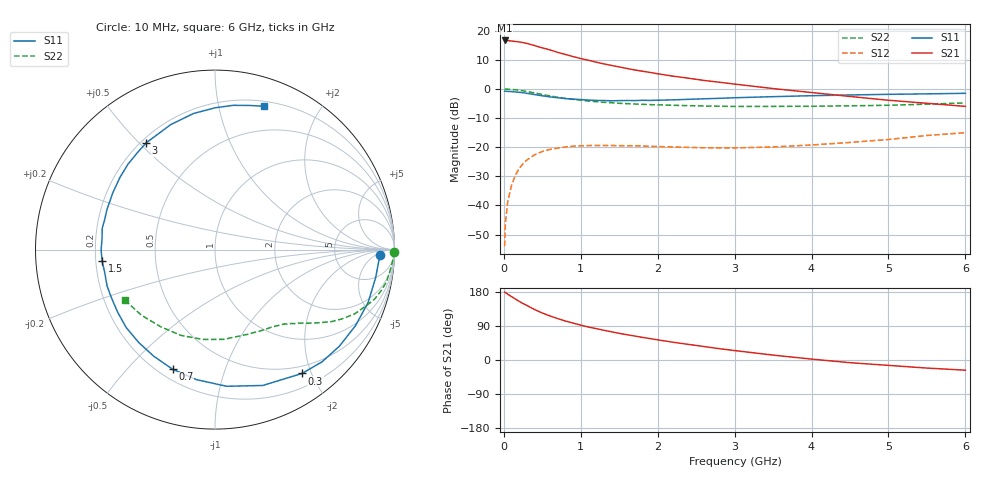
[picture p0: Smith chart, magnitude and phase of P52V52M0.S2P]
! SIEMENS Small Signal Semiconductors
! BFP183
! Si NPN RF Bipolar Junction Transistor in SOT143
! VCE = 2.5 V  IC = 2 mA
! Common Emitter S-Parameters:  March  1996
# GHz  S  MA  R  50
!  f  S11  S21  S12  S22
! GHz  MAG  ANG  MAG  ANG  MAG  ANG  MAG  ANG
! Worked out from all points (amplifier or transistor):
!   36 points, 10 MHz to 6 GHz, reference 50 ohm
!   highest |S21| = 16.7 dB at 10 MHz (marker M1)
!   |S21| within 3 dB of that: start of sweep to 565.9 MHz
!   unconditionally stable (mu >= 1): 2.092 GHz to 5.891 GHz
!   at 250 MHz: K = 0.12, MSG = 20.8 dB, |S12| = -25.7 dB
!   at 1.4 GHz: K = 0.68, MSG = 13.7 dB, |S12| = -19.4 dB
!   at 6 GHz: K = 0.98, MSG = 4.5 dB, |S12| = -15.0 dB
!   S11 on the Smith chart (normalised r, x): 10 MHz: 21, -8; 300 MHz: 0.39, -1.86; 700 MHz: 0.25, -0.68; 1.5 GHz: 0.23, -0.05; 3 GHz: 0.22, +0.52; 6 GHz: 0.25, +1.37
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0.01  0.9206 -1.8  6.819 179.0  0.002 88.4  0.999 -0.7
0.02  0.915 -3.9  6.79 178.0  0.0049 88.8  0.9934 -1.4
0.05  0.9086 -9.9  6.771 173.6  0.0115 87.8  0.9919 -3.6
0.1  0.9026 -19.0  6.672 167.3  0.0222 79.1  0.9813 -7.2
0.2  0.8776 -37.8  6.432 154.8  0.0434 68.3  0.9524 -14.1
0.25  0.8643 -46.3  6.257 148.9  0.052 64.1  0.931 -17.2
0.3  0.8434 -54.9  6.07 143.8  0.0604 59.9  0.9047 -19.8
0.4  0.8025 -70.6  5.569 133.1  0.0742 51.5  0.8569 -24.7
0.5  0.7644 -85.1  5.086 124.0  0.0845 44.4  0.8063 -28.6
0.6  0.7319 -98.1  4.699 116.2  0.0918 38.8  0.7617 -31.8
0.7  0.7074 -109.5  4.253 109.3  0.0968 33.7  0.722 -34.2
0.8  0.6848 -120.0  3.922 102.9  0.1009 29.8  0.6907 -36.3
0.9  0.6698 -129.3  3.607 97.4  0.1043 26.2  0.6647 -38.1
1.1  0.6452 -147.0  3.115 87.0  0.1068 20.7  0.6219 -41.2
1.5  0.6321 -174.2  2.393 70.3  0.1062 13.5  0.568 -46.8
1.8  0.6395 169.3  2.022 59.7  0.1051 10.8  0.5454 -51.1
2.2  0.6511 151.1  1.663 46.9  0.1011 9.4  0.5252 -57.6
3  0.7077 122.8  1.215 24.9  0.0973 13.2  0.5012 -73.2
3.5  0.7388 109.5  1.018 12.9  0.1011 17.5  0.5026 -84.3
4.5  0.7903 89.9  0.745 -7.1  0.1209 23.5  0.5143 -111.7
5.5  0.8253 76.7  0.569 -21.3  0.1592 23.6  0.5494 -138.3
6  0.8435 71.3  0.503 -26.9  0.1778 20.3  0.5761 -150.9
